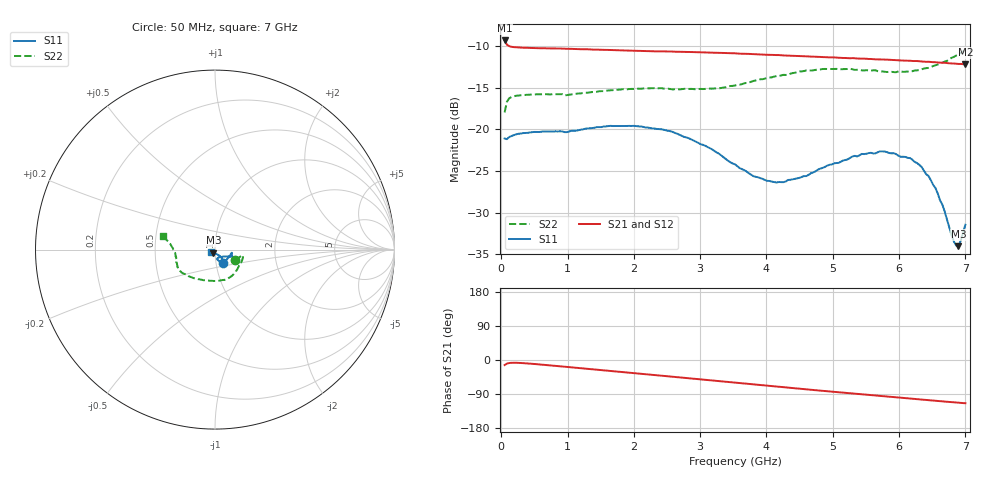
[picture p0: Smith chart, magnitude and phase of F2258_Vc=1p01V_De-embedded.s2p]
! Integrated Device Technology
! Corporate Headquarters
! 6024 Silver Creek Valley Road
! San Jose, CA 95138  USA
! Phone:  1-408-284-8200
! Toll Free:  1-800-223-1366
! Webpage:  http://www.idt.com/
! Timing and RF Division
! 515 Groton Road, Suite 102
! Westford, MA 01886-6024
! Device:  F2258
! Description: Voltage Variable RF Attenuator
! Frequency:  50.0 -  6000.00 MHz
! Package:  3x3 mm Thin QFN Plastic Package: 16 pin
! Ports:  2 RF, 2 DC
!  Pin  1  = NC
!  Pin  2  = NC
!  Pin  3  = RF2  = Port 2
!  Pin  4  = GND
!  Pin  5  = Vdd
!  Pin  6  = NC
!  Pin  7  = VCTRL
!  Pin  8  = NC
!  Pin  9  = GND
!  Pin 10  = RF1  = Port 1
!  Pin 11  = NC
!  Pin 12  = NC
!  Pin 13  = NC
!  Pin 14  = NC
!  Pin 15  = NC
!  Pin 16  = NC
! Vcntrl:  1.010 Volts
! Vdd:  +3.300 Volts
! Current:  1.156 mA
! Data:  The device was measured on a the F2258 evaluation board which has
!  individual transmission lines to the RF pins.  Data was collected
!  using a calibrated network analyzer.  The evaluation board was
!  de-embedded using a TRL calibration technique.
!  The reference plane is the edge of the package pin.
! Misc:  SN 10
!  Action Tracker AT0285
! Date Measured:  2014-12-10
! Date:  2016-01-13  MJV
! Note:
!  Integrated Device Technology supplies this data as a sample of measured
!  data at the package pin for this product.  Your particular data for this
!  product may vary.
!  Data was taken at 25 degrees C.
!  Integrated Device Technology reserves the right to change this data at anytime.
!Freq_(GHz)  S11M_(dB)  S11P_(deg)  S21M_(dB)  S21P_(deg)  S12M_(dB)  S12P_(deg)  S22M_(dB)  S22P_(deg)
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# GHz S dB R 50
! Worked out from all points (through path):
!   201 points, 50 MHz to 7 GHz, reference 50 ohm
!   highest |S21| = -9.31 dB at 50 MHz (marker M1); lowest = -12.2 dB at 7 GHz (marker M2)
!   group delay of S21, straight-line fit = 44.5 ps
!   lowest |S11| = -34.0 dB at 6.896 GHz (marker M3), VSWR 1.04, Z = 49 - j1.72 ohm
!   |S11| at or under -10 dB: start of sweep to end of sweep
!   |S22| runs from -18.0 to -10.4 dB; largest |S21 - S12| = 0.0017
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0.05  -21.09 -57.9  -9.31 -13.4  -9.32 -13.4  -17.96 -27.7
0.08475  -21.17 -31.0  -9.82 -9.5  -9.82 -9.5  -16.67 -15.2
0.189  -20.70 -14.1  -10.11 -7.3  -10.09 -7.3  -16.02 -11.4
1.2315  -19.99 -19.1  -10.37 -22.2  -10.36 -22.2  -15.63 -41.0
1.6485  -19.58 -21.3  -10.46 -28.9  -10.47 -28.9  -15.31 -52.4
2.37825  -19.97 -22.9  -10.62 -40.8  -10.61 -40.8  -15.05 -72.0
2.58675  -20.31 -24.4  -10.65 -44.2  -10.66 -44.2  -15.20 -78.1
3.07325  -21.96 -28.9  -10.75 -52.3  -10.76 -52.3  -15.14 -95.7
3.525  -24.20 -39.6  -10.85 -59.9  -10.89 -59.9  -14.72 -113.9
3.803  -25.62 -51.9  -10.95 -64.5  -10.96 -64.5  -14.18 -124.6
4.1505  -26.38 -65.5  -11.07 -70.2  -11.08 -70.2  -13.60 -135.0
4.7065  -25.16 -76.1  -11.26 -79.2  -11.28 -79.1  -12.90 -147.4
5.43625  -22.95 -66.1  -11.50 -90.5  -11.52 -90.4  -12.90 -158.7
5.85325  -22.84 -57.0  -11.63 -96.9  -11.66 -96.9  -13.08 -167.1
6.166  -23.45 -53.0  -11.75 -101.7  -11.78 -101.7  -13.07 -174.4
6.305  -24.26 -52.1  -11.82 -103.9  -11.85 -103.8  -12.87 -178.1
6.444  -25.61 -52.1  -11.87 -106.0  -11.93 -105.9  -12.61 178.4
6.54825  -27.04 -53.6  -11.92 -107.6  -11.95 -107.6  -12.30 175.5
6.6525  -29.04 -57.7  -11.97 -109.1  -12.01 -109.0  -11.99 172.8
6.82625  -33.47 -89.9  -12.08 -111.6  -12.10 -111.6  -11.29 169.0
6.89575  -34.04 -118.1  -12.13 -112.6  -12.14 -112.6  -10.93 167.5
7  -31.46 -152.7  -12.18 -114.1  -12.19 -114.1  -10.44 165.5
